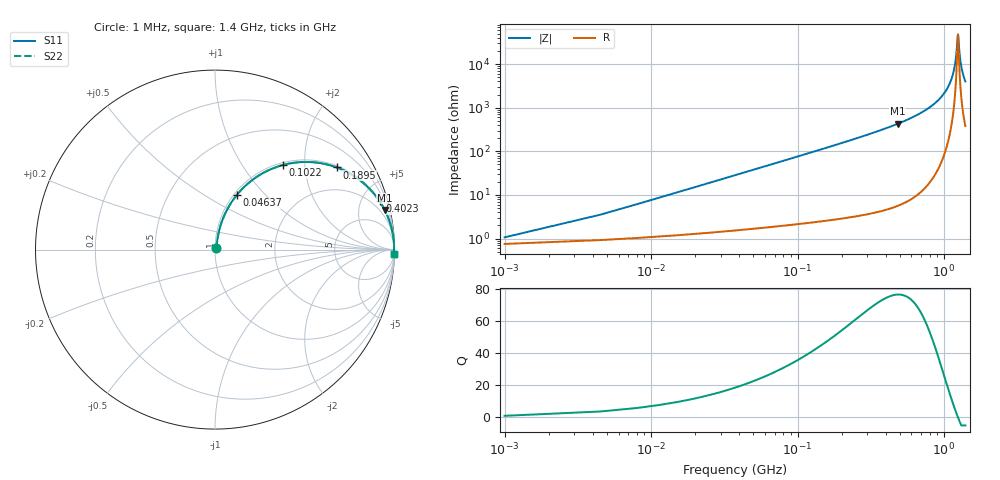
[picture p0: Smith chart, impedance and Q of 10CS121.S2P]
! Coilcraft 1008CS-121 Chip Inductor
! 02 July 2002
# MHZ S MA R 50
!Freq  MagS11  AngS11  MagS21  AngS21  MagS12  AngS12  MagS22  AngS22
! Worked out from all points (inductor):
!   402 points, 1 MHz to 1.4 GHz, reference 50 ohm
!   read as one part in series: L = 120 nH near 7.98 MHz
!   highest Q = 76.5 at 482.6 MHz (marker M1), where L = 141 nH
!   self-resonance near 1.243 GHz
!   S11 on the Smith chart (normalised r, x): 1 MHz: 1.02, +0.02; 46.37 MHz: 1.03, +0.70; 102.2 MHz: 1.04, +1.55; 189.5 MHz: 1.06, +2.92; 402.4 MHz: 1.09, +6.77; 1.4 GHz: 9, -80
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1  0.01056 44.7  0.9925 -0.4  0.9925 -0.4  0.01056 44.7
11.47  0.08593 77.8  0.9854 -4.9  0.9854 -4.9  0.08593 77.8
18.45  0.1367 77.0  0.9785 -7.8  0.9785 -7.8  0.1367 77.0
28.92  0.2108 74.2  0.964 -12.1  0.964 -12.1  0.2108 74.2
46.37  0.3261 68.3  0.9303 -19.0  0.9303 -19.0  0.3261 68.3
102.21  0.6051 51.2  0.7796 -37.2  0.7796 -37.2  0.6051 51.2
189.46  0.8183 34.0  0.5595 -54.9  0.5595 -54.9  0.8183 34.0
234.83  0.872 28.4  0.4749 -60.7  0.4749 -60.7  0.872 28.4
402.35  0.9556 16.4  0.2821 -72.8  0.2821 -72.8  0.9556 16.4
468.66  0.9688 13.6  0.2354 -75.6  0.2354 -75.6  0.9688 13.6
482.62  0.971 13.1  0.2268 -76.1  0.2268 -76.1  0.971 13.1
702.49  0.9899 7.3  0.1275 -81.8  0.1275 -81.8  0.9899 7.3
936.32  0.9963 3.5  0.06144 -84.8  0.06144 -84.8  0.9963 3.5
1079.41  0.9977 1.8  0.03063 -84.8  0.03063 -84.8  0.9977 1.8
1170.15  0.998 0.8  0.01348 -80.9  0.01348 -80.9  0.998 0.8
1205.05  0.998 0.4  0.007367 -73.8  0.007367 -73.8  0.998 0.4
1239.95  0.9979 0.1  0.002303 -26.3  0.002303 -26.3  0.9979 0.1
1246.93  0.9979 -0.0  0.002081 4.7  0.002081 4.7  0.9979 -0.0
1281.83  0.9978 -0.3  0.0064 70.2  0.0064 70.2  0.9978 -0.3
1306.26  0.9978 -0.6  0.01028 77.2  0.01028 77.2  0.9978 -0.6
1348.14  0.9976 -1.0  0.01691 81.4  0.01691 81.4  0.9976 -1.0
1400  0.9973 -1.4  0.02492 83.1  0.02492 83.1  0.9973 -1.4
